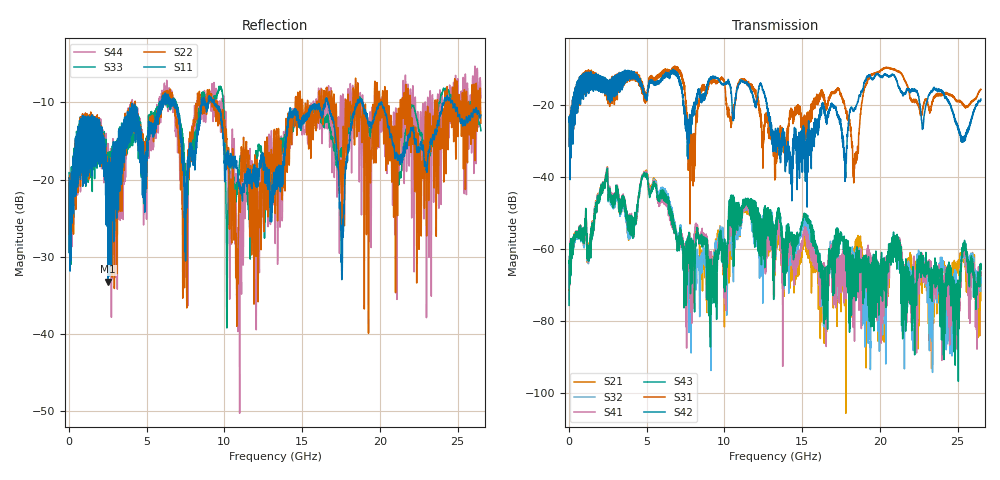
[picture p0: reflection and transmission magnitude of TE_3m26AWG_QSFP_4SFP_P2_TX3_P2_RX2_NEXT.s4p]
!Agilent Technologies,N5222A,MY51421691,A.10.00.00
!Agilent N5222A: A.10.00.00
!Date: Friday, January 30, 2015 12:35:35
!Correction: S11(Full 4 Port(1,2,3,4))
!S12(Full 4 Port(1,2,3,4))
!S13(Full 4 Port(1,2,3,4))
!S14(Full 4 Port(1,2,3,4))
!S21(Full 4 Port(1,2,3,4))
!S22(Full 4 Port(1,2,3,4))
!S23(Full 4 Port(1,2,3,4))
!S24(Full 4 Port(1,2,3,4))
!S31(Full 4 Port(1,2,3,4))
!S32(Full 4 Port(1,2,3,4))
!S33(Full 4 Port(1,2,3,4))
!S34(Full 4 Port(1,2,3,4))
!S41(Full 4 Port(1,2,3,4))
!S42(Full 4 Port(1,2,3,4))
!S43(Full 4 Port(1,2,3,4))
!S44(Full 4 Port(1,2,3,4))
!S4P File: Measurements: <S11,S12,S13,S14>,
!<S21,S22,S23,S24>,
!<S31,S32,S33,S34>,
!<S41,S42,S43,S44>:
# Hz S  dB  R 50.0
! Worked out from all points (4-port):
!   2650 points, 10 MHz to 26.5 GHz, reference 50 ohm
!   strongest paths, dB at 10 MHz, 6.63 GHz, 13.26 GHz, 19.88 GHz, 26.5 GHz:
!     S42: -24.7, -11.3, -30.4, -11.6, -18.4
!     S31: -24.9, -10.4, -34.2, -10.8, -15.7
!     S43: -75.6, -53.2, -58.9, -74.4, -65.6
!     S41: -74.1, -54.0, -62.9, -72.4, -67.2
!     S32: -70.7, -51.4, -58.8, -73.0, -71.7
!     S21: -69.1, -52.7, -61.7, -70.8, -74.3
!   lowest |S11| = -33.2 dB at 2.51 GHz (marker M1), VSWR 1.04, Z = 51 - j1.94 ohm
!   |S11| at or under -10 dB: start of sweep to 5.869 GHz; 9.353 GHz to 16.5 GHz (7.145 GHz wide, 55.3 % of centre); 20.09 GHz to 24.13 GHz (4.032 GHz wide, 18.2 % of centre)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
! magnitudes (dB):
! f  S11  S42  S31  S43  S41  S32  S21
! 10 MHz  -19.8  -24.7  -24.9  -75.6  -74.1  -70.7  -69.1
! 2.51 GHz  -33.2  -18.6  -19.7  -42.3  -41.8  -42.1  -41.6
! 9.14 GHz  -9.4  -12.9  -13.6  -78.1  -69.4  -93.7  -72.2
! 17.29 GHz  -18.0  -23.0  -15.8  -54.3  -64.2  -61.1  -72.8
! 18.39 GHz  -10.7  -21.0  -33.5  -63.2  -64.7  -62.2  -59.5
! 19.53 GHz  -12.7  -13.0  -11.7  -81.5  -78.1  -75.0  -70.1
! 26.5 GHz  -11.6  -18.4  -15.7  -65.6  -67.2  -71.7  -74.3
